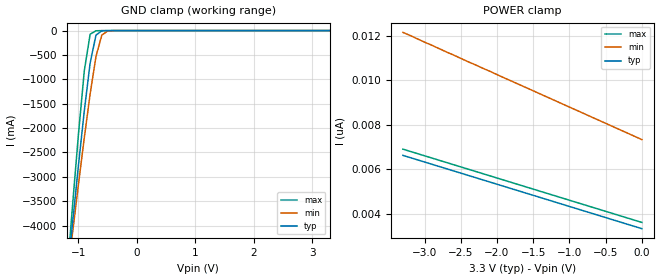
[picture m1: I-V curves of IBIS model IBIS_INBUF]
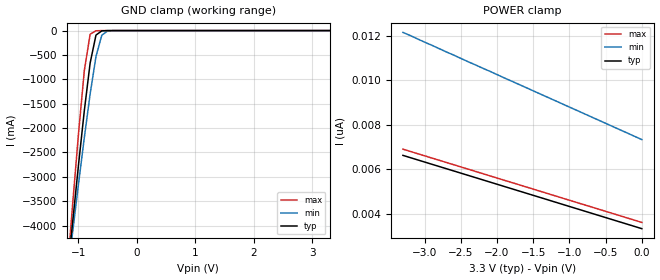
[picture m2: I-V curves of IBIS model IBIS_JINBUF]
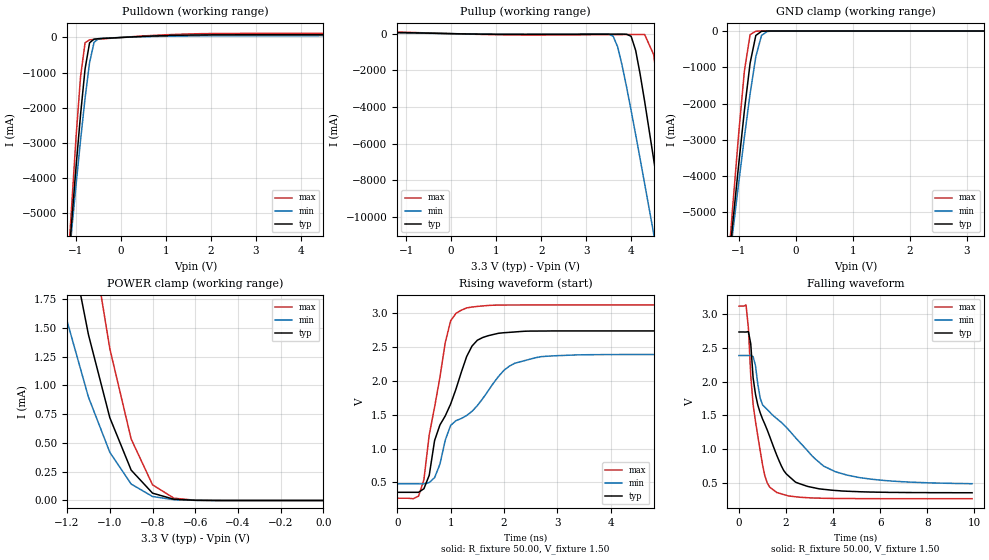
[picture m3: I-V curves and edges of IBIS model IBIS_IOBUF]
| IBIS file .ibs created by s2ibis2 version 1.1
| North Carolina State University Electronics Research Laboratory  1995
[IBIS ver]   2.1
[File name]   IDT72V73263BB.ibs
[File Rev]   1.0
[Date]   Monday, April 28, 2003
[Source]   Integrated Device Technology, Inc.
[Notes]   1. Temperatures: typ=25C, min=85C, max=-40C 2. CMOS11.5_3.3v
   process. 3. Ramp rates based on 50 ohm load.
[Disclaimer] Integrated Device Technology, Inc. ("IDT") hereby grants the
   user of this IBIS model a non-exclusive, nontransferable
   license to use this IBIS model under the following terms. The
   user is granted this license only to use the IBIS model and is
   not granted rights to sell, copy (except as needed to run the
   IBIS model), rent, lease or sub-license the IBIS model in
   whole or in part, or in modified form to anyone. The User may
   modify the IBIS model to suit its specific applications, but
   rights to derivative works and such modifications shall belong
   to IDT. This IBIS model is provided on an AS IS" basis and IDT
   makes absolutely no warranty with respect to the information
   contained herein. IDT DISCLAIMS AND CUSTOMER WAIVES ALL
   WARRANTIES, EXPRESS AND IMPLIED, INCLUDING WARRANTIES OF
   MERCHANTABILITY AND FITNESS FOR A PARTICULAR PURPOSE. THE
   ENTIRE RISK AS TO QUALITY AND PERFORMANCE IS WITH THE USER
   ACCORDINGLY, IN NO EVENT SHALL IDT BE LIABLE FOR ANY DIRECT OR
   INDIRECT DAMAGES, WHETHER IN CONTRACT OR TORT, INCLUDING ANY
   LOST PROFITS OR OTHER INCIDENTAL, CONSEQUENTIAL, EXEMPLARY, OR
   PUNITIVE DAMAGES ARISING OUT OF THE USE OR APPLICATION OF THE
   IBIS model. Further, IDT reserves the right to make changes
   without notice to any product herein to improve reliability,
   function, or design. IDT does not convey any license under
   patent rights or any other intellectual property rights,
   including those of third parties. IDT is not obligated to
   provide maintenance or support for the licensed IBIS model.
[Copyright]   Copyright 2003, Integrated Device Technology, Inc.
|   Component IDT72V73263BB
[Component]   IDT72V73263BB
[Manufacturer]   Integrated Device Technology
[Package]
| variable   typ   min   max
R_pkg   100.00m   50.00m   0.30
L_pkg   4.00nH   3.20nH   5.50nH
C_pkg   0.64pF   0.50pF   0.70pF
[Pin]  signal_name   model_name   R_pin   L_pin   C_pin
A1   C32I   IBIS_INBUF
A2   RESETB   IBIS_INBUF
A3   ODE   IBIS_INBUF
A4   RX1   IBIS_INBUF
A5   RX4   IBIS_INBUF
A6   TX0   IBIS_OUTBUF
A7   TX4   IBIS_OUTBUF
A8   TX7   IBIS_OUTBUF
A9   TX12   IBIS_OUTBUF
A10   TX15   IBIS_OUTBUF
A11   RX11   IBIS_INBUF
A12   RX15   IBIS_INBUF
A13   RX20   IBIS_INBUF
A14   TX16   IBIS_OUTBUF
A15   TX18   IBIS_OUTBUF
A16   TX19   IBIS_OUTBUF
B1   F32I   IBIS_INBUF
B2   VCC   POWER
B3   RX0   IBIS_INBUF
B4   RX2   IBIS_INBUF
B5   RX5   IBIS_INBUF
B6   TX1   IBIS_OUTBUF
B7   TX5   IBIS_OUTBUF
B8   TX8   IBIS_OUTBUF
B9   TX11   IBIS_OUTBUF
B10   TX14   IBIS_OUTBUF
B11   RX10   IBIS_INBUF
B12   RX14   IBIS_INBUF
B13   RX19   IBIS_INBUF
B14   RX23   IBIS_INBUF
B15   TX17   IBIS_OUTBUF
B16   TX20   IBIS_OUTBUF
C1   S/A   IBIS_INBUF
C2   TMS   IBIS_JINBUF
C3   TDI   IBIS_JINBUF
C4   RX3   IBIS_INBUF
C5   RX6   IBIS_INBUF
C6   TX2   IBIS_OUTBUF
C7   TX6   IBIS_OUTBUF
C8   TX9   IBIS_OUTBUF
C9   TX10   IBIS_OUTBUF
C10   TX13   IBIS_OUTBUF
C11   RX9   IBIS_INBUF
C12   RX13   IBIS_INBUF
C13   RX18   IBIS_INBUF
C14   RX22   IBIS_INBUF
C15   TX22   IBIS_OUTBUF
C16   TX21   IBIS_OUTBUF
D1   TDO   IBIS_OUTBUF
D2   TCK   IBIS_JINBUF
D3   TRSTB   IBIS_JINBUF
D4   DSB   IBIS_INBUF
D5   RX7   IBIS_INBUF
D6   TX3   IBIS_OUTBUF
D7   VCC   POWER
D8   VCC   POWER
D9   VCC   POWER
D10   VCC   POWER
D11   RX8   IBIS_INBUF
D12   RX12   IBIS_INBUF
D13   RX17   IBIS_INBUF
D14   RX21   IBIS_INBUF
D15   TX24   IBIS_OUTBUF
D16   TX23   IBIS_OUTBUF
E1   CSB   IBIS_INBUF
E2   R/WB   IBIS_INBUF
E3   A0   IBIS_INBUF
E4   A1   IBIS_INBUF
E13   RX16   IBIS_INBUF
E14   RX27   IBIS_INBUF
E15   TX26   IBIS_OUTBUF
E16   TX25   IBIS_OUTBUF
F1   A2   IBIS_INBUF
F2   A3   IBIS_INBUF
F3   A4   IBIS_INBUF
F4   A5   IBIS_INBUF
F13   TX31   IBIS_OUTBUF
F14   TX30   IBIS_OUTBUF
F15   TX29   IBIS_OUTBUF
F16   TX28   IBIS_OUTBUF
G1   A6   IBIS_INBUF
G2   A7   IBIS_INBUF
G3   A8   IBIS_INBUF
G4   VCC   POWER
G7   GND   GND
G8   GND   GND
G9   GND   GND
G10   GND   GND
G13   VCC   POWER
G14   RX26   IBIS_INBUF
G15   RX25   IBIS_INBUF
G16   RX24   IBIS_INBUF
H1   A9   IBIS_INBUF
H2   A10   IBIS_INBUF
H3   A11   IBIS_INBUF
H4   VCC   POWER
H7   GND   GND
H8   GND   GND
H9   GND   GND
H10   GND   GND
H13   VCC   POWER
H14   RX29   IBIS_INBUF
H15   RX28   IBIS_INBUF
H16   RX27   IBIS_INBUF
J1   A14   IBIS_INBUF
J2   A13   IBIS_INBUF
J3   A12   IBIS_INBUF
J4   VCC   POWER
J7   GND   GND
J8   GND   GND
J9   GND   GND
J10   GND   GND
J13   VCC   POWER
J14   RX30   IBIS_INBUF
J15   RX31   IBIS_INBUF
J16   RX32   IBIS_INBUF
K1   D15   IBIS_IOBUF
K2   DTA/BEHB   IBIS_DTABUF
K3   A15   IBIS_INBUF
K4   VCC   POWER
K7   GND   GND
K8   GND   GND
K9   GND   GND
K10   GND   GND
K13   VCC   POWER
K14   RX33   IBIS_INBUF
K15   RX34   IBIS_INBUF
K16   RX35   IBIS_INBUF
L1   D12   IBIS_IOBUF
L2   D13   IBIS_IOBUF
L3   D14   IBIS_IOBUF
L4   BELB   IBIS_INBUF
L13   RX36   IBIS_INBUF
L14   RX37   IBIS_INBUF
L15   RX38   IBIS_INBUF
L16   RX39   IBIS_INBUF
M1   D8   IBIS_IOBUF
M2   D9   IBIS_IOBUF
M3   D10   IBIS_IOBUF
M4   D11   IBIS_IOBUF
M13   TX32   IBIS_OUTBUF
M14   TX33   IBIS_OUTBUF
M15   TX34   IBIS_OUTBUF
M16   TX35   IBIS_OUTBUF
N1   D5   IBIS_IOBUF
N2   D6   IBIS_IOBUF
N3   D7   IBIS_IOBUF
N4   RX56   IBIS_INBUF
N5   TX60   IBIS_OUTBUF
N6   TX56   IBIS_OUTBUF
N7   VCC   POWER
N8   VCC   POWER
N9   VCC   POWER
N10   VCC   POWER
N11   RX51   IBIS_INBUF
N12   RX47   IBIS_INBUF
N13   TX36   IBIS_OUTBUF
N14   TX37   IBIS_OUTBUF
N15   TX38   IBIS_OUTBUF
N16   TX39   IBIS_OUTBUF
P1   D3   IBIS_IOBUF
P2   D4   IBIS_IOBUF
P3   RX60   IBIS_INBUF
P4   RX57   IBIS_INBUF
P5   TX61   IBIS_OUTBUF
P6   TX57   IBIS_OUTBUF
P7   TX53   IBIS_OUTBUF
P8   TX50   IBIS_OUTBUF
P9   TX49   IBIS_OUTBUF
P10   RX54   IBIS_INBUF
P11   RX50   IBIS_INBUF
P12   RX46   IBIS_INBUF
P13   RX43   IBIS_INBUF
P14   TX40   IBIS_OUTBUF
P15   TX41   IBIS_OUTBUF
P16   TX42   IBIS_OUTBUF
R1   D2   IBIS_IOBUF
R2   RX63   IBIS_INBUF
R3   RX61   IBIS_INBUF
R4   RX58   IBIS_INBUF
R5   TX62   IBIS_OUTBUF
R6   TX58   IBIS_OUTBUF
R7   TX54   IBIS_OUTBUF
R8   TX51   IBIS_OUTBUF
R9   TX48   IBIS_OUTBUF
R10   RX53   IBIS_INBUF
R11   RX49   IBIS_INBUF
R12   RX45   IBIS_INBUF
R13   RX42   IBIS_INBUF
R14   RX40   IBIS_INBUF
R15   TX46   IBIS_OUTBUF
R16   TX43   IBIS_OUTBUF
T1   D1   IBIS_IOBUF
T2   D0   IBIS_IOBUF
T3   RX62   IBIS_INBUF
T4   RX59   IBIS_INBUF
T5   TX63   IBIS_OUTBUF
T6   TX59   IBIS_OUTBUF
T7   TX55   IBIS_OUTBUF
T8   TX52   IBIS_OUTBUF
T9   RX55   IBIS_INBUF
T10   RX52   IBIS_INBUF
T11   RX48   IBIS_INBUF
T12   RX44   IBIS_INBUF
T13   RX41   IBIS_INBUF
T14   TX47   IBIS_OUTBUF
T15   TX45   IBIS_OUTBUF
T16   TX44   IBIS_OUTBUF
| Models and submodels in the file (5): IBIS_INBUF (Input), IBIS_JINBUF (Input), IBIS_IOBUF (I/O), IBIS_DTABUF (I/O_open_drain), IBIS_OUTBUF (Output)
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| q_o  q_o   dummy_model_0
| oe_o oe_o   dummy_model_1
| q_io q_io   dummy_model_2
| oe_iooe_io   dummy_model_3
| q_dt q_dt   dummy_model_4
| oe_dtoe_dt   dummy_model_5
|   Model IBIS_INBUF
[Model]   IBIS_INBUF
Model_type   Input
Vinl =  0.800V
Vinh =  2.000V
C_comp   3.00pF   2.00pF   4.00pF
[Temperature Range]   25.00   85.00   -40.00
[Voltage Range]   3.30V   3.00V   3.60V
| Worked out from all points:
|   GND clamp passes 1 mA (typ) near -0.51 V on its own axis
[GND_clamp]
| voltage   I(typ)   I(min)   I(max)
-3.3V     -31.65A    -27.17A    -38.32A
-1.2V     -5.139A    -5.141A    -5.07A
-1.1V     -3.937A    -4.138A    -3.57A
-1V       -2.764A    -3.154A    -2.126A
-900mV    -1.647A    -2.2A      -825mA
-800mV    -666mA     -1.301A    -74.45mA
-700mV    -92.33mA   -533mA     -4.222mA
-600mV    -6.029mA   -92.49mA   -674uA
-500mV    -245uA     -9.308mA   -69.71uA
3.3V      3.32nA     7.772nA    3.301nA
[POWER_clamp]
| voltage   I(typ)   I(min)   I(max)
-3.3V     6.621nA    12.16nA    6.901nA
-3.2V     6.521nA    12.02nA    6.801nA
-2.4V     5.721nA    10.84nA    6.001nA
0V        3.32nA     7.332nA    3.601nA
|   Model IBIS_JINBUF
[Model]   IBIS_JINBUF
Model_type   Input
Vinl =  0.800V
Vinh =  2.000V
C_comp   3.00pF   2.00pF   4.00pF
[Temperature Range]   25.00   85.00   -40.00
[Voltage Range]   3.30V   3.00V   3.60V
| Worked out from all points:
|   GND clamp passes 1 mA (typ) near -0.51 V on its own axis
[GND_clamp]
| voltage   I(typ)   I(min)   I(max)
-3.3V     -31.65A    -27.17A    -38.32A
-1.2V     -5.139A    -5.141A    -5.07A
-1.1V     -3.937A    -4.138A    -3.57A
-1V       -2.764A    -3.154A    -2.126A
-900mV    -1.647A    -2.2A      -825mA
-800mV    -666mA     -1.301A    -74.46mA
-700mV    -92.33mA   -533mA     -4.23mA
-600mV    -6.032mA   -92.49mA   -685uA
-500mV    -252uA     -9.309mA   -82.84uA
3.3V      3.32nA     7.772nA    3.301nA
[POWER_clamp]
| voltage   I(typ)   I(min)   I(max)
-3.3V     6.621nA    12.16nA    6.901nA
-3.2V     6.521nA    12.02nA    6.801nA
-2.4V     5.721nA    10.84nA    6.001nA
0V        3.32nA     7.332nA    3.601nA
|   Model IBIS_IOBUF
[Model]   IBIS_IOBUF
Model_type   I/O
Polarity   Non-Inverting
Enable   Active-High
Vinl =  0.000V
Vinh =  3.300V
Vmeas =  1.500V
Cref = 30.000pF
Rref = 50.000
Vref =  1.500V
C_comp   3.00pF   2.00pF   4.00pF
[Temperature Range]   25.00   85.00   -40.00
[Voltage Range]   3.30V   3.00V   3.60V
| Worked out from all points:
|   slope of the pulldown table from 0 to 0.495 V, typ, clamps not added: 16.1 ohm
|   slope of the pullup table from 0 to 0.495 V, typ, clamps not added: 22.5 ohm
|   GND clamp passes 1 mA (typ) near -0.51 V on its own axis
|   POWER clamp passes 1 mA (typ) near -1.04 V on its own axis
|   rising waveform, R_fixture 50.00, V_fixture 1.50: 20-80 % time 614ps typ, 1.01ns min, 352ps max; typ from 0.355 V to 2.73 V
|   falling waveform, R_fixture 50.00, V_fixture 1.50: 20-80 % time 1.14ns typ, 2.41ns min, 534ps max; typ from 2.73 V to 0.356 V
[Pulldown]
| voltage   I(typ)   I(min)   I(max)
-3.3V     -42.01A    -36.04A    -50.9A
-1.5V     -11.71A    -10.89A    -12.87A
-1V       -3.67A     -4.184A    -2.828A
-900mV    -2.19A     -2.919A    -1.111A
-800mV    -893.8mA   -1.729A    -150.1mA
-700mV    -151.7mA   -712.3mA   -66.27mA
-600mV    -46.32mA   -137.9mA   -55.05mA
-500mV    -34.57mA   -33.69mA   -46mA
-400mV    -27.67mA   -20.5mA    -37.18mA
1.5V      67.91mA    43.34mA    99.95mA
4.7V      84.5mA     56.12mA    122mA
6.6V      131mA      78.82mA    191mA
[Pullup]
| voltage   I(typ)   I(min)   I(max)
-3.3V     37.98mA    18.68mA    52.21mA
3.5V      -28.52mA   -25.74mA   -54.78mA
3.6V      -27.26mA   -136mA     -53.29mA
3.7V      -26.03mA   -719mA     -51.79mA
4V        -146mA     -4.196A    -47.34mA
4.1V      -906mA     -5.501A    -45.99mA
4.3V      -3.69A     -8.178A    -48.94mA
4.5V      -6.84A     -10.9A     -1.138A
4.7V      -10.09A    -13.65A    -4.78A
4.9V      -13.39A    -16.42A    -8.799A
5.1V      -16.72A    -19.21A    -12.91A
6.6V      -42.01A    -40.27A    -44.53A
[GND_clamp]
| voltage   I(typ)   I(min)   I(max)
-3.3V     -42.01A    -36.04A    -50.9A
-1.2V     -6.817A    -6.818A    -6.727A
-1.1V     -5.222A    -5.488A    -4.737A
-1V       -3.667A    -4.183A    -2.82A
-900mV    -2.185A    -2.917A    -1.095A
-800mV    -883mA     -1.726A    -98.49mA
-700mV    -122mA     -706mA     -5.285mA
-600mV    -7.89mA    -122mA     -799uA
-500mV    -309uA     -12.24mA   -81.59uA
3.3V      3.324nA    12.74nA    3.301nA
[POWER_clamp]
| voltage   I(typ)   I(min)   I(max)
-3.3V     37.81mA    12.13mA    58.7mA
-1.3V     3.527mA    2.369mA    5.591mA
-1.2V     2.39mA     1.56mA     3.898mA
-1.1V     1.442mA    899uA      2.459mA
-1V       720uA      419uA      1.32mA
-900mV    264uA      143uA      534uA
-800mV    63.73uA    34.5uA     136uA
-700mV    10.82uA    6.689uA    20.13uA
-600mV    1.552uA    1.171uA    2.049uA
0V        3.324nA    8.566nA    3.601nA
[Ramp]
| variable   typ   min   max
dV/dt_r   1.24/0.79n   0.81/1.43n   1.61/0.43n
dV/dt_f   1.46/1.39n   1.11/2.63n   1.74/0.72n
R_load = 50.00
[Rising Waveform]
R_fixture = 50.00
V_fixture = 1.50
C_fixture = 0.000F
| time   V(typ)   V(min)   V(max)
0s        355mV      480mV      268mV
400ps     355mV      480mV      299mV
500ps     408mV      479mV      541mV
600ps     607mV      499mV      1.204V
700ps     1.118V     571mV      1.61V
1ns       1.654V     1.34V      2.879V
1.3ns     2.354V     1.486V     3.07V
2ns       2.705V     2.153V     3.112V
2.7ns     2.73V      2.353V     3.114V
9.9ns     2.731V     2.383V     3.114V
[Falling Waveform]
R_fixture = 50.00
V_fixture = 1.50
C_fixture = 0.000F
| time   V(typ)   V(min)   V(max)
0s        2.732V     2.384V     3.114V
300ps     2.731V     2.384V     3.132V
500ps     2.556V     2.386V     2.086V
600ps     2.055V     2.368V     1.662V
900ps     1.539V     1.755V     980mV
1.3ns     1.192V     1.55V      441mV
2ns       638mV      1.327V     319mV
2.9ns     451mV      982mV      283mV
4.6ns     378mV      616mV      270mV
9.9ns     356mV      490mV      268mV
